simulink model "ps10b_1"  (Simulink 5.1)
settings: Solver=ode45  StartTime=0.0  StopTime=10.0  RelTol=1e-3

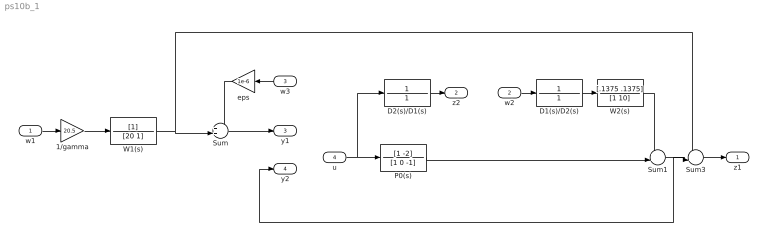
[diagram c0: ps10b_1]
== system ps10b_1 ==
  w1 : Inport
  w2 : Inport  Port=2
  w3 : Inport  Orientation=left  Port=3
  u : Inport  Port=4
  1/gamma : Gain  Gain=20.5
  D1(s)/D2(s) : TransferFcn  Numerator=1  Denominator=1
  D2(s)/D1(s) : TransferFcn  Numerator=1  Denominator=1
  P0(s) : TransferFcn  Numerator=[1 -2]  Denominator=[1 0 -1]
  Sum : Sum  Inputs=++|
  Sum1 : Sum  Inputs=++|
  Sum3 : Sum  Inputs=-+|
  W1(s) : TransferFcn  Denominator=[20 1]
  W2(s) : TransferFcn  Numerator=[.1375 .1375]  Denominator=[1 10]
  eps : Gain  Orientation=left  Gain=1e-6
  z1 : Outport
  z2 : Outport  Port=2
  y1 : Outport  Port=3
  y2 : Outport  Port=4
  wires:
  1/gamma/1 -> W1(s)/1
  W1(s)/1 -> Sum/2, Sum3/1
  eps/1 -> Sum/1
  w3/1 -> eps/1
  Sum/1 -> y1/1
  u/1 -> P0(s)/1, D2(s)/D1(s)/1
  D2(s)/D1(s)/1 -> z2/1
  w2/1 -> D1(s)/D2(s)/1
  D1(s)/D2(s)/1 -> W2(s)/1
  W2(s)/1 -> Sum1/1
  P0(s)/1 -> Sum1/2
  Sum1/1 -> Sum3/2, y2/1
  Sum3/1 -> z1/1
  w1/1 -> 1/gamma/1
